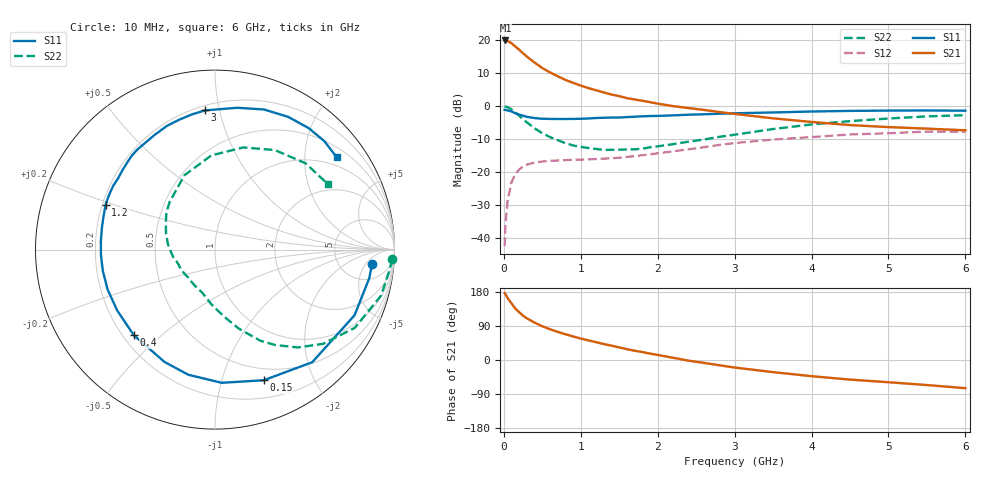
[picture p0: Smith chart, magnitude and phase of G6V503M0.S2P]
! SIEMENS Small Signal Semiconductors
! BFG193
! Si NPN RF Bipolar Junction Transistor in SOT223
! VCE = 0.5 V  IC = 3 mA
! Common Emitter S-Parameters:  August  1996
# GHz  S  MA  R  50
!  f  S11  S21  S12  S22
! GHz  MAG  ANG  MAG  ANG  MAG  ANG  MAG  ANG
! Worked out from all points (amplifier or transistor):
!   36 points, 10 MHz to 6 GHz, reference 50 ohm
!   highest |S21| = 20.0 dB at 20 MHz (marker M1)
!   |S21| within 3 dB of that: start of sweep to 208 MHz
!   unconditionally stable (mu >= 1): 1.209 GHz to end of sweep
!   at 250 MHz: K = 0.26, MSG = 17.2 dB, |S12| = -18.4 dB
!   at 1.4 GHz: K = 1.11, MAG = 7.7 dB, |S12| = -15.9 dB
!   at 6 GHz: K = 1.03, MAG = -0.8 dB, |S12| = -7.8 dB
!   S11 on the Smith chart (normalised r, x): 10 MHz: 10, -7; 150 MHz: 0.37, -1.37; 400 MHz: 0.24, -0.41; 1.2 GHz: 0.21, +0.19; 3 GHz: 0.23, +0.91; 6 GHz: 0.75, +2.80
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0.01  0.8786 -5.3  9.917 176.5  0.0074 89.9  0.9878 -3.1
0.02  0.8742 -10.5  9.962 174.1  0.015 86.3  0.9804 -6.3
0.05  0.8592 -25.2  9.752 163.0  0.0373 74.7  0.9605 -15.4
0.1  0.829 -49.2  9.035 149.4  0.0694 63.9  0.8928 -29.2
0.15  0.7769 -69.5  8.045 135.6  0.0929 53.2  0.7989 -41.1
0.2  0.7431 -87.1  7.193 125.9  0.109 45.7  0.7139 -49.8
0.25  0.713 -102.0  6.355 116.9  0.1205 39.1  0.6269 -57.9
0.3  0.6863 -114.2  5.648 109.8  0.1287 34.7  0.5653 -63.7
0.4  0.6573 -133.5  4.585 98.6  0.1384 27.8  0.459 -73.3
0.5  0.6418 -148.1  3.789 89.0  0.1434 22.9  0.3863 -81.0
0.6  0.6383 -159.6  3.252 81.2  0.1468 20.2  0.3381 -87.7
0.7  0.6361 -169.1  2.844 74.2  0.1487 18.3  0.303 -94.2
0.9  0.6378 175.7  2.257 62.1  0.153 15.8  0.2519 -105.9
1.1  0.6481 163.4  1.875 51.7  0.1547 15.0  0.2302 -119.0
1.2  0.6592 157.6  1.739 47.0  0.1567 14.9  0.223 -125.4
1.6  0.68 139.1  1.321 28.6  0.1688 15.3  0.219 -151.3
2.2  0.7222 117.7  0.999 5.9  0.2048 13.8  0.2636 173.7
3  0.7775 94.0  0.761 -19.9  0.274 4.3  0.3669 133.5
3.5  0.7999 81.1  0.651 -32.0  0.3097 -6.8  0.4481 112.3
4.5  0.8446 61.1  0.514 -51.7  0.3699 -25.7  0.5907 74.5
5.5  0.8581 44.8  0.454 -66.1  0.4097 -48.7  0.6973 43.6
6  0.8513 37.1  0.428 -74.4  0.4091 -61.7  0.7277 29.9
